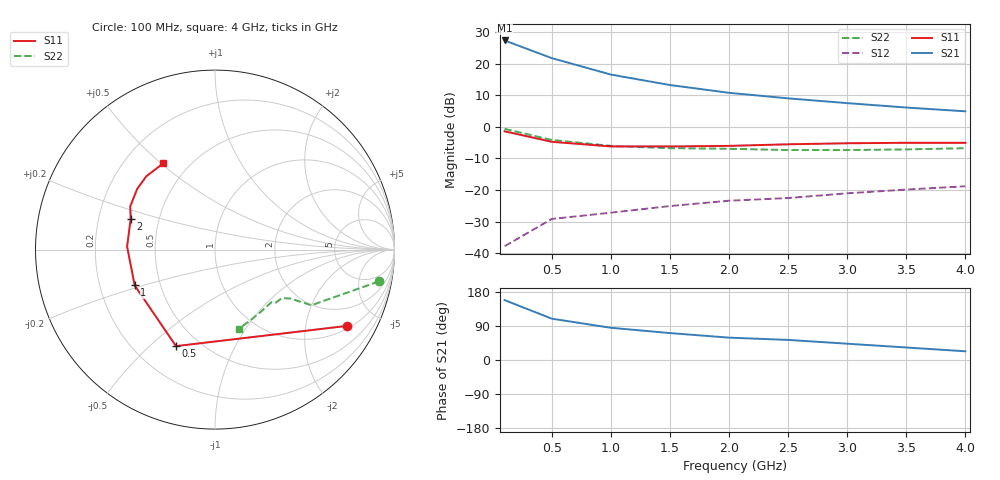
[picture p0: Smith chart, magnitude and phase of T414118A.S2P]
!AT-41411
!S AND NOISE PARAMETERS at Vce=8V  Ic=10mA.  LAST UPDATED 07-21-92
# ghz s ma r 50
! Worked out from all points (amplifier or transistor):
!   9 points, 100 MHz to 4 GHz, reference 50 ohm
!   highest |S21| = 27.3 dB at 100 MHz (marker M1)
!   |S21| within 3 dB of that: start of sweep to 314.4 MHz
!   unconditionally stable (mu >= 1): 1.217 GHz to end of sweep
!   at 500 MHz: K = 0.54, MSG = 25.4 dB, |S12| = -29.1 dB
!   at 2 GHz: K = 1.17, MAG = 14.5 dB, |S12| = -23.3 dB
!   at 4 GHz: K = 1.20, MAG = 9.1 dB, |S12| = -18.8 dB
!   lowest NFmin = 1.30 dB at 100 MHz
!   S11 on the Smith chart (normalised r, x): 100 MHz: 1.11, -3.40; 500 MHz: 0.37, -0.61; 1 GHz: 0.36, -0.19; 2 GHz: 0.34, +0.16; 4 GHz: 0.36, +0.51
0.1  0.85 -30.0  23.2 158.0  0.013 64.0  0.93 -11.0
0.5  0.58 -112.0  12.18 109.0  0.035 44.0  0.62 -30.0
1  0.49 -156.0  6.7 85.0  0.044 43.0  0.5 -33.0
1.5  0.49 178.0  4.58 71.0  0.056 47.0  0.46 -36.0
2  0.5 160.0  3.45 59.0  0.068 47.0  0.45 -41.0
2.5  0.53 153.0  2.82 53.0  0.075 56.0  0.43 -43.0
3  0.55 142.0  2.37 43.0  0.089 54.0  0.43 -53.0
3.5  0.56 133.0  2.02 33.0  0.102 52.0  0.44 -63.0
4  0.56 121.0  1.76 23.0  0.115 49.0  0.46 -73.0
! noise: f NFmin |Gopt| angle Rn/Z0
0.1  1.3  0.12  4  0.17
0.5  1.3  0.1  23  0.17
1  1.4  0.07  57  0.16
2  1.8  0.09  -158  0.16
4  3.5  0.31  -87  0.38
